| This Model is valid for Automotive grade 2 Temperature Range -40C<=Tc<=105C
| Valid for LPDDR4-4266 operation
| Part Number   VDD/VDDQ   Package   Architecture
| SCE11U64324EF-04ZA2   1.1 +0.07/-0.04  FBGA   2G bit x 32 (200b,QDP,10x14.5x1.1)
| SCE11U32322EF-04ZA2   1.1 +0.07/-0.04  FBGA   1G bit x 32 (200b,DDP,10x14.5x1.1)
[IBIS Ver]  5.0
[File Name] usesnxx32ea2.ibs
[Date]   05/20/2025
[File Rev]  1.0
[Source] Simulation of a silicon level SPICE model
[Notes]  IBIS Characteristics for I/O Buffer
  IBIS Model Revision History: Rev 2.0:
  2026-03-27 - IBIS model file PN number change
[Disclaimer]  The IBIS models are for modeling purpose only and are subject to change without any notice. UniIC is not
  responsible for any problems the models may cause.
[Copyright] Copyright 2025 UniIC Semiconductors Corp. All rights reserved
|   Component SCE11U64324EF-04ZA2
[Component] SCE11U64324EF-04ZA2
[Manufacturer] UniIC Semiconductors Corp.
[Package]
|   typ   min   max
R_pkg   1781.0m   683.00m   3347.0m
L_pkg   3.313nH   1.222nH   6.060nH
C_pkg   1.150pF   0.604pF   2.030pF
[Pin] signal_name  model_name   R_pin   L_pin   C_pin
A1   DNU   NC
A2   DNU   NC
A3   VSS   GND
A4   VDD2   POWER
A5   ZQ0   NC
A8   ZQ1   NC
A9   VDD2   POWER
A10   VSS   GND
A11   DNU   NC
A12   DNU   NC
B1   DNU   NC
B2   DQ0_A   DQ   892.22m   1.783nH   0.667pF
B3   VDDQ   POWER
B4   DQ7_A   DQ   942.05m   1.831nH   0.712pF
B5   VDDQ   POWER
B8   VDDQ   POWER
B9   DQ15_A   DQ   905.71m   1.724nH   0.652pF
B10   VDDQ   POWER
B11   DQ8_A   DQ   951.20m   1.847nH   0.708pF
B12   DNU   NC
C1   VSS   GND
C2   DQ1_A   DQ   869.40m   1.675nH   0.663pF
C3   DMI0_A   DQ   802.20m   1.539nH   0.644pF
C4   DQ6_A   DQ   695.07m   1.386nH   0.604pF
C5   VSS   GND
C8   VSS   GND
C9   DQ14_A   DQ   809.80m   1.568nH   0.657pF
C10   DMI1_A   DQ   843.49m   1.585nH   0.669pF
C11   DQ9_A   DQ   862.40m   1.663nH   0.667pF
C12   VSS   GND
D1   VDDQ   POWER
D2   VSS   GND
D3   DQS0_t_A   DQS   872.77m   1.603nH   0.663pF
D4   VSS   GND
D5   VDDQ   POWER
D8   VDDQ   POWER
D9   VSS   GND
D10   DQS1_t_A   DQS   906.95m   1.659nH   0.687pF
D11   VSS   GND
D12   VDDQ   POWER
E1   VSS   GND
E2   DQ2_A   DQ   766.79m   1.410nH   0.641pF
E3   DQS0_c_A   DQS   892.70m   1.616nH   0.682pF
E4   DQ5_A   DQ   683.10m   1.243nH   0.617pF
E5   VSS   GND
E8   VSS   GND
E9   DQ13_A   DQ   751.68m   1.328nH   0.636pF
E10   DQS1_c_A   DQS   932.00m   1.697nH   0.709pF
E11   DQ10_A   DQ   805.68m   1.499nH   0.658pF
E12   VSS   GND
F1   VDD1   POWER
F2   DQ3_A   DQ   815.20m   1.487nH   0.658pF
F3   VDDQ   POWER
F4   DQ4_A   DQ   684.70m   1.222nH   0.624pF
F5   VDD2   POWER
F8   VDD2   POWER
F9   DQ12_A   DQ   754.00m   1.333nH   0.665pF
F10   VDDQ   POWER
F11   DQ11_A   DQ   816.75m   1.527nH   0.656pF
F12   VDD1   POWER
G1   VSS   GND
G2   ODT_CA_A   ODTCA_INPUT   3223.0m   5.380nH   0.839pF
G3   VSS   GND
G4   VDD1   POWER
G5   VSS   GND
G8   VSS   GND
G9   VDD1   POWER
G10   VSS   GND
G11   NC   NC
G12   VSS   GND
H1   VDD2   POWER
H2   CA0_A   CA_INPUT   1381.0m   2.440nH   0.952pF
H3   CS1_A   CS_INPUT
H4   CS0_A   CS_INPUT
H5   VDD2   POWER
H8   VDD2   POWER
H9   CA2_A   CA_INPUT   1146.0m   2.055nH   0.856pF
H10   CA3_A   CA_INPUT   1283.0m   2.280nH   0.920pF
H11   CA4_A   CA_INPUT   1456.0m   2.590nH   1.005pF
H12   VDD2   POWER
J1   VSS   GND
J2   CA1_A   CA_INPUT   1531.0m   2.640nH   1.061pF
J3   VSS   GND
J4   CKE0_A   CKE_INPUT
J5   CKE1_A   CKE_INPUT
J8   CK_t_A   CLK_INPUT   1327.0m   2.423nH   0.917pF
J9   CK_c_A   CLK_INPUT   1352.0m   2.460nH   0.936pF
J10   VSS   GND
J11   CA5_A   CA_INPUT   1682.0m   2.901nH   1.080pF
J12   VSS   GND
K1   VDD2   POWER
K2   VSS   GND
K3   VDD2   POWER
K4   VSS   GND
K5   NC   NC
K8   NC   NC
K9   VSS   GND
K10   VDD2   POWER
K11   VSS   GND
K12   VDD2   POWER
N1   VDD2   POWER
N2   VSS   GND
N3   VDD2   POWER
N4   VSS   GND
N5   NC   NC
N8   NC   NC
N9   VSS   GND
N10   VDD2   POWER
N11   VSS   GND
N12   VDD2   POWER
P1   VSS   GND
P2   CA1_B   CA_INPUT   2001.0m   3.590nH   1.240pF
P3   VSS   GND
P4   CKE0_B   CKE_INPUT
P5   CKE1_B   CKE_INPUT
P8   CK_t_B   CLK_INPUT   1908.0m   3.371nH   1.215pF
P9   CK_c_B   CLK_INPUT   1352.0m   2.464nH   0.936pF
P10   VSS   GND
P11   CA5_B   CA_INPUT   1935.0m   3.552nH   1.192pF
P12   VSS   GND
R1   VDD2   POWER
R2   CA0_B   CA_INPUT   2110.0m   3.790nH   1.283pF
R3   CS1_B   CS_INPUT
R4   CS0_B   CS_INPUT
R5   VDD2   POWER
R8   VDD2   POWER
R9   CA2_B   CA_INPUT   1965.0m   3.398nH   1.229pF
R10   CA3_B   CA_INPUT   2061.0m   3.706nH   1.260pF
R11   CA4_B   CA_INPUT   1859.0m   3.388nH   1.151pF
R12   VDD2   POWER
T1   VSS   GND
T2   ODT_CA_B   ODTCA_INPUT   1974.0m   3.548nH   1.128pF
T3   VSS   GND
T4   VDD1   POWER
T5   VSS   GND
T8   VSS   GND
T9   VDD1   POWER
T10   VSS   GND
T11   RESET_n   NC
T12   VSS   GND
U1   VDD1   POWER
U2   DQ3_B   DQ   2687.0m   4.766nH   1.558pF
U3   VDDQ   POWER
U4   DQ4_B   DQ   2425.0m   4.233nH   1.469pF
U5   VDD2   POWER
U8   VDD2   POWER
U9   DQ12_B   DQ   3116.0m   5.207nH   1.812pF
U10   VDDQ   POWER
U11   DQ11_B   DQ   3179.0m   5.321nH   1.828pF
U12   VDD1   POWER
V1   VSS   GND
V2   DQ2_B   DQ   2588.0m   4.551nH   1.513pF
V3   DQS0_c_B   DQS   2438.0m   4.346nH   1.466pF
V4   DQ5_B   DQ   2290.0m   4.012nH   1.391pF
V5   VSS   GND
V8   VSS   GND
V9   DQ13_B   DQ   3013.0m   5.038nH   1.759pF
V10   DQS1_c_B   DQS   3073.0m   5.198nH   1.833pF
V11   DQ10_B   DQ   3240.0m   5.404nH   1.898pF
V12   VSS   GND
W1   VDDQ   POWER
W2   VSS   GND
W3   DQS0_t_B   DQS   2438.0m   4.346nH   1.466pF
W4   VSS   GND
W5   VDDQ   POWER
W8   VDDQ   POWER
W9   VSS   GND
W10   DQS1_t_B   DQS   3167.0m   5.386nH   1.871pF
W11   VSS   GND
W12   VDDQ   POWER
Y1   VSS   GND
Y2   DQ1_B   DQ   2484.0m   4.410nH   1.467pF
Y3   DMI0_B   DQ   2282.0m   4.056nH   1.378pF
Y4   DQ6_B   DQ   2149.0m   3.822nH   1.313pF
Y5   VSS   GND
Y8   VSS   GND
Y9   DQ14_B   DQ   3051.0m   5.183nH   1.804pF
Y10   DMI1_B   DQ   3195.0m   5.155nH   1.899pF
Y11   DQ9_B   DQ   3347.0m   5.680nH   1.932pF
Y12   VSS   GND
AA1   DNU   NC
AA2   DQ0_B   DQ   2472.0m   4.484nH   1.453pF
AA3   VDDQ   POWER
AA4   DQ7_B   DQ   2196.0m   4.004nH   1.284pF
AA5   VDDQ   POWER
AA8   VDDQ   POWER
AA9   DQ15_B   DQ   3046.0m   5.081nH   1.820pF
AA10  VDDQ   POWER
AA11  DQ8_B   DQ   3565.0m   6.060nH   2.037pF
AA12  DNU   NC
AB1   DNU   NC
AB2   DNU   NC
AB3   VSS   GND
AB4   VDD2   POWER
AB5   VSS   GND
AB8   VSS   GND
AB9   VDD2   POWER
AB10  VSS   GND
AB11  DNU   NC
AB12  DNU   NC
[Diff Pin]  inv_pin  vdiff   tdelay_typ   tdelay_min   tdelay_max
D3   E3   0.120V   0.000s   NA   NA
W3   V3   0.120V   0.000s   NA   NA
D10   E10   0.120V   0.000s   NA   NA
W10   V10   0.120V   0.000s   NA   NA
J8   J9   0.145V   0.000s   NA   NA
P8   P9   0.145V   0.000s   NA   NA
|   Component SCE11U32322EF-04ZA2
[Component] SCE11U32322EF-04ZA2
[Manufacturer] UniIC Semiconductors Corp.
[Package]
|   typ   min   max
R_pkg   1781.0m   683.00m   3340.0m
L_pkg   3.313nH   1.222nH   6.060nH
C_pkg   1.150pF   0.604pF   2.030pF
[Pin] signal_name  model_name   R_pin   L_pin   C_pin
A1   DNU   NC
A2   DNU   NC
A3   VSS   GND
A4   VDD2   POWER
A5   ZQ0   NC
A8   ZQ1   NC
A9   VDD2   POWER
A10   VSS   GND
A11   DNU   NC
A12   DNU   NC
B1   DNU   NC
B2   DQ0_A   DQ   892.22m   1.783nH   0.667pF
B3   VDDQ   POWER
B4   DQ7_A   DQ   942.05m   1.831nH   0.712pF
B5   VDDQ   POWER
B8   VDDQ   POWER
B9   DQ15_A   DQ   905.71m   1.724nH   0.652pF
B10   VDDQ   POWER
B11   DQ8_A   DQ   951.20m   1.847nH   0.708pF
B12   DNU   NC
C1   VSS   GND
C2   DQ1_A   DQ   869.40m   1.675nH   0.663pF
C3   DMI0_A   DQ   802.20m   1.539nH   0.644pF
C4   DQ6_A   DQ   695.07m   1.386nH   0.604pF
C5   VSS   GND
C8   VSS   GND
C9   DQ14_A   DQ   809.80m   1.568nH   0.657pF
C10   DMI1_A   DQ   843.49m   1.585nH   0.669pF
C11   DQ9_A   DQ   862.40m   1.663nH   0.667pF
C12   VSS   GND
D1   VDDQ   POWER
D2   VSS   GND
D3   DQS0_t_A   DQS   872.77m   1.603nH   0.663pF
D4   VSS   GND
D5   VDDQ   POWER
D8   VDDQ   POWER
D9   VSS   GND
D10   DQS1_t_A   DQS   906.95m   1.659nH   0.687pF
D11   VSS   GND
D12   VDDQ   POWER
E1   VSS   GND
E2   DQ2_A   DQ   766.79m   1.410nH   0.641pF
E3   DQS0_c_A   DQS   892.70m   1.616nH   0.682pF
E4   DQ5_A   DQ   683.10m   1.243nH   0.617pF
E5   VSS   GND
E8   VSS   GND
E9   DQ13_A   DQ   751.68m   1.328nH   0.636pF
E10   DQS1_c_A   DQS   932.00m   1.697nH   0.709pF
E11   DQ10_A   DQ   805.68m   1.499nH   0.658pF
E12   VSS   GND
F1   VDD1   POWER
F2   DQ3_A   DQ   815.20m   1.487nH   0.658pF
F3   VDDQ   POWER
F4   DQ4_A   DQ   684.70m   1.222nH   0.624pF
F5   VDD2   POWER
F8   VDD2   POWER
F9   DQ12_A   DQ   754.00m   1.333nH   0.665pF
F10   VDDQ   POWER
F11   DQ11_A   DQ   816.75m   1.527nH   0.656pF
F12   VDD1   POWER
G1   VSS   GND
G2   ODT_CA_A   ODTCA_INPUT   3223.0m   5.380nH   0.839pF
G3   VSS   GND
G4   VDD1   POWER
G5   VSS   GND
G8   VSS   GND
G9   VDD1   POWER
G10   VSS   GND
G11   NC   NC
G12   VSS   GND
H1   VDD2   POWER
H2   CA0_A   CA_INPUT   1381.0m   2.440nH   0.952pF
H3   NC   NC
H4   CS0_A   CS_INPUT
H5   VDD2   POWER
H8   VDD2   POWER
H9   CA2_A   CA_INPUT   1146.0m   2.055nH   0.856pF
H10   CA3_A   CA_INPUT   1283.0m   2.280nH   0.920pF
H11   CA4_A   CA_INPUT   1456.0m   2.590nH   1.005pF
H12   VDD2   POWER
J1   VSS   GND
J2   CA1_A   CA_INPUT   1531.0m   2.640nH   1.061pF
J3   VSS   GND
J4   CKE0_A   CKE_INPUT
J5   NC   NC
J8   CK_t_A   CLK_INPUT   1327.0m   2.423nH   0.917pF
J9   CK_c_A   CLK_INPUT   1352.0m   2.460nH   0.936pF
J10   VSS   GND
J11   CA5_A   CA_INPUT   1682.0m   2.901nH   1.080pF
J12   VSS   GND
K1   VDD2   POWER
K2   VSS   GND
K3   VDD2   POWER
K4   VSS   GND
K5   NC   NC
K8   NC   NC
K9   VSS   GND
K10   VDD2   POWER
K11   VSS   GND
K12   VDD2   POWER
N1   VDD2   POWER
N2   VSS   GND
N3   VDD2   POWER
N4   VSS   GND
N5   NC   NC
N8   NC   NC
N9   VSS   GND
N10   VDD2   POWER
N11   VSS   GND
N12   VDD2   POWER
P1   VSS   GND
P2   CA1_B   CA_INPUT   2001.0m   3.590nH   1.240pF
P3   VSS   GND
P4   CKE0_B   CKE_INPUT
P5   NC   NC
P8   CK_t_B   CLK_INPUT   1908.0m   3.371nH   1.215pF
P9   CK_c_B   CLK_INPUT   1352.0m   2.464nH   0.936pF
P10   VSS   GND
P11   CA5_B   CA_INPUT   1935.0m   3.552nH   1.192pF
P12   VSS   GND
R1   VDD2   POWER
R2   CA0_B   CA_INPUT   2110.0m   3.790nH   1.283pF
R3   NC   NC
R4   CS0_B   CS_INPUT
R5   VDD2   POWER
R8   VDD2   POWER
R9   CA2_B   CA_INPUT   1965.0m   3.398nH   1.229pF
R10   CA3_B   CA_INPUT   2061.0m   3.706nH   1.260pF
R11   CA4_B   CA_INPUT   1859.0m   3.388nH   1.151pF
R12   VDD2   POWER
T1   VSS   GND
T2   ODT_CA_B   ODTCA_INPUT   1974.0m   3.548nH   1.128pF
T3   VSS   GND
T4   VDD1   POWER
T5   VSS   GND
T8   VSS   GND
T9   VDD1   POWER
T10   VSS   GND
T11   RESET_n   NC
T12   VSS   GND
U1   VDD1   POWER
U2   DQ3_B   DQ   2687.0m   4.766nH   1.558pF
U3   VDDQ   POWER
U4   DQ4_B   DQ   2425.0m   4.233nH   1.469pF
U5   VDD2   POWER
U8   VDD2   POWER
U9   DQ12_B   DQ   3116.0m   5.207nH   1.812pF
U10   VDDQ   POWER
U11   DQ11_B   DQ   3179.0m   5.321nH   1.828pF
U12   VDD1   POWER
V1   VSS   GND
V2   DQ2_B   DQ   2588.0m   4.551nH   1.513pF
V3   DQS0_c_B   DQS   2438.0m   4.346nH   1.466pF
V4   DQ5_B   DQ   2290.0m   4.012nH   1.391pF
V5   VSS   GND
V8   VSS   GND
V9   DQ13_B   DQ   3013.0m   5.038nH   1.759pF
V10   DQS1_c_B   DQS   3073.0m   5.198nH   1.833pF
V11   DQ10_B   DQ   3240.0m   5.404nH   1.898pF
V12   VSS   GND
W1   VDDQ   POWER
W2   VSS   GND
W3   DQS0_t_B   DQS   2438.0m   4.346nH   1.466pF
W4   VSS   GND
W5   VDDQ   POWER
W8   VDDQ   POWER
W9   VSS   GND
W10   DQS1_t_B   DQS   3167.0m   5.386nH   1.871pF
W11   VSS   GND
W12   VDDQ   POWER
Y1   VSS   GND
Y2   DQ1_B   DQ   2484.0m   4.410nH   1.467pF
Y3   DMI0_B   DQ   2282.0m   4.056nH   1.378pF
Y4   DQ6_B   DQ   2149.0m   3.822nH   1.313pF
Y5   VSS   GND
Y8   VSS   GND
Y9   DQ14_B   DQ   3051.0m   5.183nH   1.804pF
Y10   DMI1_B   DQ   3195.0m   5.155nH   1.899pF
Y11   DQ9_B   DQ   3347.0m   5.680nH   1.932pF
Y12   VSS   GND
AA1   DNU   NC
AA2   DQ0_B   DQ   2472.0m   4.484nH   1.453pF
AA3   VDDQ   POWER
AA4   DQ7_B   DQ   2196.0m   4.004nH   1.284pF
AA5   VDDQ   POWER
AA8   VDDQ   POWER
AA9   DQ15_B   DQ   3046.0m   5.081nH   1.820pF
AA10  VDDQ   POWER
AA11  DQ8_B   DQ   356.05m   6.060nH   2.037pF
AA12  DNU   NC
AB1   DNU   NC
AB2   DNU   NC
AB3   VSS   GND
AB4   VDD2   POWER
AB5   VSS   GND
AB8   VSS   GND
AB9   VDD2   POWER
AB10  VSS   GND
AB11  DNU   NC
AB12  DNU   NC
[Diff Pin]  inv_pin  vdiff   tdelay_typ   tdelay_min   tdelay_max
D3   E3   0.120V   0.000s   NA   NA
W3   V3   0.120V   0.000s   NA   NA
D10   E10   0.120V   0.000s   NA   NA
W10   V10   0.120V   0.000s   NA   NA
J8   J9   0.145V   0.000s   NA   NA
P8   P9   0.145V   0.000s   NA   NA
|   Model Selector
[Model Selector] DQ
| Data I/O models
DQ_PD40_SOC-ODT40_VOH30_4266   40 Ohm Pulldown, 40 Ohm System ODT Setting, VOH=VDDQ/3.0, 3200-4266Mbps
DQ_PD40_SOC-ODT48_VOH30_4266   40 Ohm Pulldown, 48 Ohm System ODT Setting, VOH=VDDQ/3.0, 3200-4266Mbps
DQ_PD40_SOC-ODT60_VOH30_4266   40 Ohm Pulldown, 60 Ohm System ODT Setting, VOH=VDDQ/3.0, 3200-4266Mbps
DQ_PD40_SOC-ODT80_VOH30_4266   40 Ohm Pulldown, 80 Ohm System ODT Setting, VOH=VDDQ/3.0, 3200-4266Mbps
DQ_PD40_SOC-ODT120_VOH30_4266   40 Ohm Pulldown, 120 Ohm System ODT Setting, VOH=VDDQ/3.0, 3200-4266Mbps
DQ_PD40_SOC-ODT240_VOH30_4266   40 Ohm Pulldown, 240 Ohm System ODT Setting, VOH=VDDQ/3.0, 3200-4266Mbps
DQ_PD40_SOC-ODTDIS_VOH30_4266   40 Ohm Pulldown, SOC ODT disabled setting, VOH=VDDQ/3.0 cal. point, 3200-4266Mbps
DQ_PD40_SOC-ODT80_VOH25_4266   40 Ohm Pulldown, 80 Ohm System ODT Setting, VOH=VDDQ/2.5, 3200-4266Mbps
DQ_PD40_SOC-ODT120_VOH25_4266   40 Ohm Pulldown, 120 Ohm System ODT Setting, VOH=VDDQ/2.5, 3200-4266Mbps
DQ_PD40_SOC-ODT240_VOH25_4266   40 Ohm Pulldown, 240 Ohm System ODT Setting, VOH=VDDQ/2.5, 3200-4266Mbps
DQ_PD40_SOC-ODTDIS_VOH25_4266   40 Ohm Pulldown, SOC ODT disabled setting, VOH=VDDQ/2.5 cal. point, 3200-4266Mbps
DQ_PD48_SOC-ODT40_VOH30_4266   48 Ohm Pulldown, 40 Ohm System ODT Setting, VOH=VDDQ/3.0, 3200-4266Mbps
DQ_PD48_SOC-ODT48_VOH30_4266   48 Ohm Pulldown, 48 Ohm System ODT Setting, VOH=VDDQ/3.0, 3200-4266Mbps
DQ_PD48_SOC-ODT60_VOH30_4266   48 Ohm Pulldown, 60 Ohm System ODT Setting, VOH=VDDQ/3.0, 3200-4266Mbps
DQ_PD48_SOC-ODT80_VOH30_4266   48 Ohm Pulldown, 80 Ohm System ODT Setting, VOH=VDDQ/3.0, 3200-4266Mbps
DQ_PD48_SOC-ODT120_VOH30_4266   48 Ohm Pulldown, 120 Ohm System ODT Setting, VOH=VDDQ/3.0, 3200-4266Mbps
DQ_PD48_SOC-ODT240_VOH30_4266   48 Ohm Pulldown, 240 Ohm System ODT Setting, VOH=VDDQ/3.0, 3200-4266Mbps
DQ_PD48_SOC-ODTDIS_VOH30_4266   48 Ohm Pulldown, SOC ODT disabled setting, VOH=VDDQ/3.0 cal. point, 3200-4266Mbps
DQ_PD48_SOC-ODT80_VOH25_4266   48 Ohm Pulldown, 80 Ohm System ODT Setting, VOH=VDDQ/2.5, 3200-4266Mbps
DQ_PD48_SOC-ODT120_VOH25_4266   48 Ohm Pulldown, 120 Ohm System ODT Setting, VOH=VDDQ/2.5, 3200-4266Mbps
DQ_PD48_SOC-ODT240_VOH25_4266   48 Ohm Pulldown, 240 Ohm System ODT Setting, VOH=VDDQ/2.5, 3200-4266Mbps
DQ_PD48_SOC-ODTDIS_VOH25_4266   48 Ohm Pulldown, SOC ODT disabled setting, VOH=VDDQ/2.5 cal. point, 3200-4266Mbps
DQ_PD60_SOC-ODT40_VOH30_4266   60 Ohm Pulldown, 40 Ohm System ODT Setting, VOH=VDDQ/3.0, 3200-4266Mbps
DQ_PD60_SOC-ODT48_VOH30_4266   60 Ohm Pulldown, 48 Ohm System ODT Setting, VOH=VDDQ/3.0, 3200-4266Mbps
DQ_PD60_SOC-ODT60_VOH30_4266   60 Ohm Pulldown, 60 Ohm System ODT Setting, VOH=VDDQ/3.0, 3200-4266Mbps
DQ_PD60_SOC-ODT80_VOH30_4266   60 Ohm Pulldown, 80 Ohm System ODT Setting, VOH=VDDQ/3.0, 3200-4266Mbps
DQ_PD60_SOC-ODT120_VOH30_4266   60 Ohm Pulldown, 120 Ohm System ODT Setting, VOH=VDDQ/3.0, 3200-4266Mbps
DQ_PD60_SOC-ODT240_VOH30_4266   60 Ohm Pulldown, 240 Ohm System ODT Setting, VOH=VDDQ/3.0, 3200-4266Mbps
DQ_PD60_SOC-ODTDIS_VOH30_4266   60 Ohm Pulldown, SOC ODT disabled setting, VOH=VDDQ/3.0 cal. point, 3200-4266Mbps
DQ_PD60_SOC-ODT80_VOH25_4266   60 Ohm Pulldown, 80 Ohm System ODT Setting, VOH=VDDQ/2.5, 3200-4266Mbps
DQ_PD60_SOC-ODT120_VOH25_4266   60 Ohm Pulldown, 120 Ohm System ODT Setting, VOH=VDDQ/2.5, 3200-4266Mbps
DQ_PD60_SOC-ODT240_VOH25_4266   60 Ohm Pulldown, 240 Ohm System ODT Setting, VOH=VDDQ/2.5, 3200-4266Mbps
DQ_PD60_SOC-ODTDIS_VOH25_4266   60 Ohm Pulldown, SOC ODT disabled setting, VOH=VDDQ/2.5 cal. point, 3200-4266Mbps
DQ_PD80_SOC-ODT40_VOH30_4266   80 Ohm Pulldown, 40 Ohm System ODT Setting, VOH=VDDQ/3.0, 3200-4266Mbps
DQ_PD80_SOC-ODT48_VOH30_4266   80 Ohm Pulldown, 48 Ohm System ODT Setting, VOH=VDDQ/3.0, 3200-4266Mbps
DQ_PD80_SOC-ODT60_VOH30_4266   80 Ohm Pulldown, 60 Ohm System ODT Setting, VOH=VDDQ/3.0, 3200-4266Mbps
DQ_PD80_SOC-ODT80_VOH30_4266   80 Ohm Pulldown, 80 Ohm System ODT Setting, VOH=VDDQ/3.0, 3200-4266Mbps
DQ_PD80_SOC-ODT120_VOH30_4266   80 Ohm Pulldown, 120 Ohm System ODT Setting, VOH=VDDQ/3.0, 3200-4266Mbps
DQ_PD80_SOC-ODT240_VOH30_4266   80 Ohm Pulldown, 240 Ohm System ODT Setting, VOH=VDDQ/3.0, 3200-4266Mbps
DQ_PD80_SOC-ODTDIS_VOH30_4266   80 Ohm Pulldown, SOC ODT disabled setting, VOH=VDDQ/3.0 cal. point, 3200-4266Mbps
DQ_PD80_SOC-ODT80_VOH25_4266   80 Ohm Pulldown, 80 Ohm System ODT Setting, VOH=VDDQ/2.5, 3200-4266Mbps
DQ_PD80_SOC-ODT120_VOH25_4266   80 Ohm Pulldown, 120 Ohm System ODT Setting, VOH=VDDQ/2.5, 3200-4266Mbps
DQ_PD80_SOC-ODT240_VOH25_4266   80 Ohm Pulldown, 240 Ohm System ODT Setting, VOH=VDDQ/2.5, 3200-4266Mbps
DQ_PD80_SOC-ODTDIS_VOH25_4266   80 Ohm Pulldown, SOC ODT disabled setting, VOH=VDDQ/2.5 cal. point, 3200-4266Mbps
DQ_PD120_SOC-ODT40_VOH30_4266   120 Ohm Pulldown, 40 Ohm System ODT Setting, VOH=VDDQ/3.0, 3200-4266Mbps
DQ_PD120_SOC-ODT48_VOH30_4266   120 Ohm Pulldown, 48 Ohm System ODT Setting, VOH=VDDQ/3.0, 3200-4266Mbps
DQ_PD120_SOC-ODT60_VOH30_4266   120 Ohm Pulldown, 60 Ohm System ODT Setting, VOH=VDDQ/3.0, 3200-4266Mbps
DQ_PD120_SOC-ODT80_VOH30_4266   120 Ohm Pulldown, 80 Ohm System ODT Setting, VOH=VDDQ/3.0, 3200-4266Mbps
DQ_PD120_SOC-ODT120_VOH30_4266  120 Ohm Pulldown, 120 Ohm System ODT Setting, VOH=VDDQ/3.0, 3200-4266Mbps
DQ_PD120_SOC-ODT240_VOH30_4266  120 Ohm Pulldown, 240 Ohm System ODT Setting, VOH=VDDQ/3.0, 3200-4266Mbps
DQ_PD120_SOC-ODTDIS_VOH30_4266  120 Ohm Pulldown, SOC ODT disabled setting, VOH=VDDQ/3.0 cal. point, 3200-4266Mbps
DQ_PD120_SOC-ODT80_VOH25_4266   120 Ohm Pulldown, 80 Ohm System ODT Setting, VOH=VDDQ/2.5, 3200-4266Mbps
DQ_PD120_SOC-ODT120_VOH25_4266  120 Ohm Pulldown, 120 Ohm System ODT Setting, VOH=VDDQ/2.5, 3200-4266Mbps
DQ_PD120_SOC-ODT240_VOH25_4266  120 Ohm Pulldown, 240 Ohm System ODT Setting, VOH=VDDQ/2.5, 3200-4266Mbps
DQ_PD120_SOC-ODTDIS_VOH25_4266  120 Ohm Pulldown, SOC ODT disabled setting, VOH=VDDQ/2.5 cal. point, 3200-4266Mbps
DQ_PD240_SOC-ODT40_VOH30_4266   240 Ohm Pulldown, 40 Ohm System ODT Setting, VOH=VDDQ/3.0, 3200-4266Mbps
DQ_PD240_SOC-ODT48_VOH30_4266   240 Ohm Pulldown, 48 Ohm System ODT Setting, VOH=VDDQ/3.0, 3200-4266Mbps
DQ_PD240_SOC-ODT60_VOH30_4266   240 Ohm Pulldown, 60 Ohm System ODT Setting, VOH=VDDQ/3.0, 3200-4266Mbps
DQ_PD240_SOC-ODT80_VOH30_4266   240 Ohm Pulldown, 80 Ohm System ODT Setting, VOH=VDDQ/3.0, 3200-4266Mbps
DQ_PD240_SOC-ODT120_VOH30_4266  240 Ohm Pulldown, 120 Ohm System ODT Setting, VOH=VDDQ/3.0, 3200-4266Mbps
DQ_PD240_SOC-ODT240_VOH30_4266  240 Ohm Pulldown, 240 Ohm System ODT Setting, VOH=VDDQ/3.0, 3200-4266Mbps
DQ_PD240_SOC-ODTDIS_VOH30_4266  240 Ohm Pulldown, SOC ODT disabled setting, VOH=VDDQ/3.0 cal. point, 3200-4266Mbps
DQ_PD240_SOC-ODT80_VOH25_4266   240 Ohm Pulldown, 80 Ohm System ODT Setting, VOH=VDDQ/2.5, 3200-4266Mbps
DQ_PD240_SOC-ODT120_VOH25_4266  240 Ohm Pulldown, 120 Ohm System ODT Setting, VOH=VDDQ/2.5, 3200-4266Mbps
DQ_PD240_SOC-ODT240_VOH25_4266  240 Ohm Pulldown, 240 Ohm System ODT Setting, VOH=VDDQ/2.5, 3200-4266Mbps
DQ_PD240_SOC-ODTDIS_VOH25_4266  240 Ohm Pulldown, SOC ODT disabled setting, VOH=VDDQ/2.5 cal. point, 3200-4266Mbps
DQ_IN_ODTOFF_4266   with no ODT, 3200-4266Mbps
DQ_IN_ODT40_4266   with 40ohm ODT, 3200-4266Mbps
DQ_IN_ODT48_4266   with 48ohm ODT, 3200-4266Mbps
DQ_IN_ODT60_4266   with 60ohm ODT, 3200-4266Mbps
DQ_IN_ODT80_4266   with 80ohm ODT, 3200-4266Mbps
DQ_IN_ODT120_4266   with 120ohm ODT, 3200-4266Mbps
DQ_IN_ODT240_4266   with 240ohm ODT, 3200-4266Mbps
[Model Selector] DQS
| Data Strobe I/O models
DQS_PD40_SOC-ODT40_VOH30_4266   40 Ohm Pulldown, 40 Ohm System ODT Setting, VOH=VDDQ/3.0, 3200-4266Mbps
DQS_PD40_SOC-ODT48_VOH30_4266   40 Ohm Pulldown, 48 Ohm System ODT Setting, VOH=VDDQ/3.0, 3200-4266Mbps
DQS_PD40_SOC-ODT60_VOH30_4266   40 Ohm Pulldown, 60 Ohm System ODT Setting, VOH=VDDQ/3.0, 3200-4266Mbps
DQS_PD40_SOC-ODT80_VOH30_4266   40 Ohm Pulldown, 80 Ohm System ODT Setting, VOH=VDDQ/3.0, 3200-4266Mbps
DQS_PD40_SOC-ODT120_VOH30_4266  40 Ohm Pulldown, 120 Ohm System ODT Setting, VOH=VDDQ/3.0, 3200-4266Mbps
DQS_PD40_SOC-ODT240_VOH30_4266  40 Ohm Pulldown, 240 Ohm System ODT Setting, VOH=VDDQ/3.0, 3200-4266Mbps
DQS_PD40_SOC-ODTDIS_VOH30_4266  40 Ohm Pulldown, SOC ODT disabled setting, VOH=VDDQ/3.0 cal. point, 3200-4266Mbps
DQS_PD40_SOC-ODT80_VOH25_4266   40 Ohm Pulldown, 80 Ohm System ODT Setting, VOH=VDDQ/2.5, 3200-4266Mbps
DQS_PD40_SOC-ODT120_VOH25_4266  40 Ohm Pulldown, 120 Ohm System ODT Setting, VOH=VDDQ/2.5, 3200-4266Mbps
DQS_PD40_SOC-ODT240_VOH25_4266  40 Ohm Pulldown, 240 Ohm System ODT Setting, VOH=VDDQ/2.5, 3200-4266Mbps
DQS_PD40_SOC-ODTDIS_VOH25_4266  40 Ohm Pulldown, SOC ODT disabled setting, VOH=VDDQ/2.5 cal. point, 3200-4266Mbps
DQS_PD48_SOC-ODT40_VOH30_4266   48 Ohm Pulldown, 40 Ohm System ODT Setting, VOH=VDDQ/3.0, 3200-4266Mbps
DQS_PD48_SOC-ODT48_VOH30_4266   48 Ohm Pulldown, 48 Ohm System ODT Setting, VOH=VDDQ/3.0, 3200-4266Mbps
DQS_PD48_SOC-ODT60_VOH30_4266   48 Ohm Pulldown, 60 Ohm System ODT Setting, VOH=VDDQ/3.0, 3200-4266Mbps
DQS_PD48_SOC-ODT80_VOH30_4266   48 Ohm Pulldown, 80 Ohm System ODT Setting, VOH=VDDQ/3.0, 3200-4266Mbps
DQS_PD48_SOC-ODT120_VOH30_4266  48 Ohm Pulldown, 120 Ohm System ODT Setting, VOH=VDDQ/3.0, 3200-4266Mbps
DQS_PD48_SOC-ODT240_VOH30_4266  48 Ohm Pulldown, 240 Ohm System ODT Setting, VOH=VDDQ/3.0, 3200-4266Mbps
DQS_PD48_SOC-ODTDIS_VOH30_4266  48 Ohm Pulldown, SOC ODT disabled setting, VOH=VDDQ/3.0 cal. point, 3200-4266Mbps
DQS_PD48_SOC-ODT80_VOH25_4266   48 Ohm Pulldown, 80 Ohm System ODT Setting, VOH=VDDQ/2.5, 3200-4266Mbps
DQS_PD48_SOC-ODT120_VOH25_4266  48 Ohm Pulldown, 120 Ohm System ODT Setting, VOH=VDDQ/2.5, 3200-4266Mbps
DQS_PD48_SOC-ODT240_VOH25_4266  48 Ohm Pulldown, 240 Ohm System ODT Setting, VOH=VDDQ/2.5, 3200-4266Mbps
DQS_PD48_SOC-ODTDIS_VOH25_4266  48 Ohm Pulldown, SOC ODT disabled setting, VOH=VDDQ/2.5 cal. point, 3200-4266Mbps
DQS_PD60_SOC-ODT40_VOH30_4266   60 Ohm Pulldown, 40 Ohm System ODT Setting, VOH=VDDQ/3.0, 3200-4266Mbps
DQS_PD60_SOC-ODT48_VOH30_4266   60 Ohm Pulldown, 48 Ohm System ODT Setting, VOH=VDDQ/3.0, 3200-4266Mbps
DQS_PD60_SOC-ODT60_VOH30_4266   60 Ohm Pulldown, 60 Ohm System ODT Setting, VOH=VDDQ/3.0, 3200-4266Mbps
DQS_PD60_SOC-ODT80_VOH30_4266   60 Ohm Pulldown, 80 Ohm System ODT Setting, VOH=VDDQ/3.0, 3200-4266Mbps
DQS_PD60_SOC-ODT120_VOH30_4266  60 Ohm Pulldown, 120 Ohm System ODT Setting, VOH=VDDQ/3.0, 3200-4266Mbps
DQS_PD60_SOC-ODT240_VOH30_4266  60 Ohm Pulldown, 240 Ohm System ODT Setting, VOH=VDDQ/3.0, 3200-4266Mbps
DQS_PD60_SOC-ODTDIS_VOH30_4266  60 Ohm Pulldown, SOC ODT disabled setting, VOH=VDDQ/3.0 cal. point, 3200-4266Mbps
DQS_PD60_SOC-ODT80_VOH25_4266   60 Ohm Pulldown, 80 Ohm System ODT Setting, VOH=VDDQ/2.5, 3200-4266Mbps
DQS_PD60_SOC-ODT120_VOH25_4266  60 Ohm Pulldown, 120 Ohm System ODT Setting, VOH=VDDQ/2.5, 3200-4266Mbps
DQS_PD60_SOC-ODT240_VOH25_4266  60 Ohm Pulldown, 240 Ohm System ODT Setting, VOH=VDDQ/2.5, 3200-4266Mbps
DQS_PD60_SOC-ODTDIS_VOH25_4266  60 Ohm Pulldown, SOC ODT disabled setting, VOH=VDDQ/2.5 cal. point, 3200-4266Mbps
DQS_PD80_SOC-ODT40_VOH30_4266   80 Ohm Pulldown, 40 Ohm System ODT Setting, VOH=VDDQ/3.0, 3200-4266Mbps
DQS_PD80_SOC-ODT48_VOH30_4266   80 Ohm Pulldown, 48 Ohm System ODT Setting, VOH=VDDQ/3.0, 3200-4266Mbps
DQS_PD80_SOC-ODT60_VOH30_4266   80 Ohm Pulldown, 60 Ohm System ODT Setting, VOH=VDDQ/3.0, 3200-4266Mbps
DQS_PD80_SOC-ODT80_VOH30_4266   80 Ohm Pulldown, 80 Ohm System ODT Setting, VOH=VDDQ/3.0, 3200-4266Mbps
DQS_PD80_SOC-ODT120_VOH30_4266  80 Ohm Pulldown, 120 Ohm System ODT Setting, VOH=VDDQ/3.0, 3200-4266Mbps
DQS_PD80_SOC-ODT240_VOH30_4266  80 Ohm Pulldown, 240 Ohm System ODT Setting, VOH=VDDQ/3.0, 3200-4266Mbps
DQS_PD80_SOC-ODTDIS_VOH30_4266  80 Ohm Pulldown, SOC ODT disabled setting, VOH=VDDQ/3.0 cal. point, 3200-4266Mbps
DQS_PD80_SOC-ODT80_VOH25_4266   80 Ohm Pulldown, 80 Ohm System ODT Setting, VOH=VDDQ/2.5, 3200-4266Mbps
DQS_PD80_SOC-ODT120_VOH25_4266  80 Ohm Pulldown, 120 Ohm System ODT Setting, VOH=VDDQ/2.5, 3200-4266Mbps
DQS_PD80_SOC-ODT240_VOH25_4266  80 Ohm Pulldown, 240 Ohm System ODT Setting, VOH=VDDQ/2.5, 3200-4266Mbps
DQS_PD80_SOC-ODTDIS_VOH25_4266  80 Ohm Pulldown, SOC ODT disabled setting, VOH=VDDQ/2.5 cal. point, 3200-4266Mbps
DQS_PD120_SOC-ODT40_VOH30_4266  120 Ohm Pulldown, 40 Ohm System ODT Setting, VOH=VDDQ/3.0, 3200-4266Mbps
DQS_PD120_SOC-ODT48_VOH30_4266  120 Ohm Pulldown, 48 Ohm System ODT Setting, VOH=VDDQ/3.0, 3200-4266Mbps
DQS_PD120_SOC-ODT60_VOH30_4266  120 Ohm Pulldown, 60 Ohm System ODT Setting, VOH=VDDQ/3.0, 3200-4266Mbps
DQS_PD120_SOC-ODT80_VOH30_4266  120 Ohm Pulldown, 80 Ohm System ODT Setting, VOH=VDDQ/3.0, 3200-4266Mbps
DQS_PD120_SOC-ODT120_VOH30_4266 120 Ohm Pulldown, 120 Ohm System ODT Setting, VOH=VDDQ/3.0, 3200-4266Mbps
DQS_PD120_SOC-ODT240_VOH30_4266 120 Ohm Pulldown, 240 Ohm System ODT Setting, VOH=VDDQ/3.0, 3200-4266Mbps
DQS_PD120_SOC-ODTDIS_VOH30_4266 120 Ohm Pulldown, SOC ODT disabled setting, VOH=VDDQ/3.0 cal. point, 3200-4266Mbps
DQS_PD120_SOC-ODT80_VOH25_4266  120 Ohm Pulldown, 80 Ohm System ODT Setting, VOH=VDDQ/2.5, 3200-4266Mbps
DQS_PD120_SOC-ODT120_VOH25_4266 120 Ohm Pulldown, 120 Ohm System ODT Setting, VOH=VDDQ/2.5, 3200-4266Mbps
DQS_PD120_SOC-ODT240_VOH25_4266 120 Ohm Pulldown, 240 Ohm System ODT Setting, VOH=VDDQ/2.5, 3200-4266Mbps
DQS_PD120_SOC-ODTDIS_VOH25_4266 120 Ohm Pulldown, SOC ODT disabled setting, VOH=VDDQ/2.5 cal. point, 3200-4266Mbps
DQS_PD240_SOC-ODT40_VOH30_4266  240 Ohm Pulldown, 40 Ohm System ODT Setting, VOH=VDDQ/3.0, 3200-4266Mbps
DQS_PD240_SOC-ODT48_VOH30_4266  240 Ohm Pulldown, 48 Ohm System ODT Setting, VOH=VDDQ/3.0, 3200-4266Mbps
DQS_PD240_SOC-ODT60_VOH30_4266  240 Ohm Pulldown, 60 Ohm System ODT Setting, VOH=VDDQ/3.0, 3200-4266Mbps
DQS_PD240_SOC-ODT80_VOH30_4266  240 Ohm Pulldown, 80 Ohm System ODT Setting, VOH=VDDQ/3.0, 3200-4266Mbps
DQS_PD240_SOC-ODT120_VOH30_4266 240 Ohm Pulldown, 120 Ohm System ODT Setting, VOH=VDDQ/3.0, 3200-4266Mbps
DQS_PD240_SOC-ODT240_VOH30_4266 240 Ohm Pulldown, 240 Ohm System ODT Setting, VOH=VDDQ/3.0, 3200-4266Mbps
DQS_PD240_SOC-ODTDIS_VOH30_4266 240 Ohm Pulldown, SOC ODT disabled setting, VOH=VDDQ/3.0 cal. point, 3200-4266Mbps
DQS_PD240_SOC-ODT80_VOH25_4266  240 Ohm Pulldown, 80 Ohm System ODT Setting, VOH=VDDQ/2.5, 3200-4266Mbps
DQS_PD240_SOC-ODT120_VOH25_4266 240 Ohm Pulldown, 120 Ohm System ODT Setting, VOH=VDDQ/2.5, 3200-4266Mbps
DQS_PD240_SOC-ODT240_VOH25_4266 240 Ohm Pulldown, 240 Ohm System ODT Setting, VOH=VDDQ/2.5, 3200-4266Mbps
DQS_PD240_SOC-ODTDIS_VOH25_4266 240 Ohm Pulldown, SOC ODT disabled setting, VOH=VDDQ/2.5 cal. point, 3200-4266Mbps
DQS_IN_ODTOFF_4266   with no ODT, 3200-4266Mbps
DQS_IN_ODT40_4266   with 40ohm ODT, 3200-4266Mbps
DQS_IN_ODT48_4266   with 48ohm ODT, 3200-4266Mbps
DQS_IN_ODT60_4266   with 60ohm ODT, 3200-4266Mbps
DQS_IN_ODT80_4266   with 80ohm ODT, 3200-4266Mbps
DQS_IN_ODT120_4266   with 120ohm ODT, 3200-4266Mbps
DQS_IN_ODT240_4266   with 240ohm ODT, 3200-4266Mbps
[Model Selector] CA_INPUT
| CA Input models
CA_INPUT_ODTOFF_4266   with no ODT, 3200-4266Mbps
CA_INPUT_ODT40_4266   with 40ohm ODT, 3200-4266Mbps
CA_INPUT_ODT48_4266   with 48ohm ODT, 3200-4266Mbps
CA_INPUT_ODT60_4266   with 60ohm ODT, 3200-4266Mbps
CA_INPUT_ODT80_4266   with 80ohm ODT, 3200-4266Mbps
CA_INPUT_ODT120_4266   with 120ohm ODT, 3200-4266Mbps
CA_INPUT_ODT240_4266   with 240ohm ODT, 3200-4266Mbps
[Model Selector] CS_INPUT
| CS Input models
CS_INPUT_ODTOFF_4266   with no ODT, 3200-4266Mbps
CS_INPUT_ODT40_4266   with 40ohm ODT, 3200-4266Mbps
CS_INPUT_ODT48_4266   with 48ohm ODT, 3200-4266Mbps
CS_INPUT_ODT60_4266   with 60ohm ODT, 3200-4266Mbps
CS_INPUT_ODT80_4266   with 80ohm ODT, 3200-4266Mbps
CS_INPUT_ODT120_4266   with 120ohm ODT, 3200-4266Mbps
CS_INPUT_ODT240_4266   with 240ohm ODT, 3200-4266Mbps
[Model Selector] CLK_INPUT
| Clock Input models
CLK_INPUT_ODTOFF_4266   with no ODT, 3200-4266Mbps
CLK_INPUT_ODT40_4266   with 40ohm ODT, 3200-4266Mbps
CLK_INPUT_ODT48_4266   with 48ohm ODT, 3200-4266Mbps
CLK_INPUT_ODT60_4266   with 60ohm ODT, 3200-4266Mbps
CLK_INPUT_ODT80_4266   with 80ohm ODT, 3200-4266Mbps
CLK_INPUT_ODT120_4266   with 120ohm ODT, 3200-4266Mbps
CLK_INPUT_ODT240_4266   with 240ohm ODT, 3200-4266Mbps
| Models and submodels in the file (175): DQ_PD40_SOC-ODT40_VOH30_4266 (I/O), DQ_PD40_SOC-ODT48_VOH30_4266 (I/O), DQ_PD40_SOC-ODT60_VOH30_4266 (I/O), DQ_PD40_SOC-ODT80_VOH30_4266 (I/O), DQ_PD40_SOC-ODT120_VOH30_4266 (I/O), DQ_PD40_SOC-ODT240_VOH30_4266 (I/O), DQ_PD40_SOC-ODTDIS_VOH30_4266 (I/O), DQ_PD40_SOC-ODT80_VOH25_4266 (I/O), DQ_PD40_SOC-ODT120_VOH25_4266 (I/O), DQ_PD40_SOC-ODT240_VOH25_4266 (I/O), DQ_PD40_SOC-ODTDIS_VOH25_4266 (I/O), DQ_PD48_SOC-ODT40_VOH30_4266 (I/O), DQ_PD48_SOC-ODT48_VOH30_4266 (I/O), DQ_PD48_SOC-ODT60_VOH30_4266 (I/O), DQ_PD48_SOC-ODT80_VOH30_4266 (I/O), DQ_PD48_SOC-ODT120_VOH30_4266 (I/O), DQ_PD48_SOC-ODT240_VOH30_4266 (I/O), DQ_PD48_SOC-ODTDIS_VOH30_4266 (I/O), DQ_PD48_SOC-ODT80_VOH25_4266 (I/O), DQ_PD48_SOC-ODT120_VOH25_4266 (I/O), DQ_PD48_SOC-ODT240_VOH25_4266 (I/O), DQ_PD48_SOC-ODTDIS_VOH25_4266 (I/O), DQ_PD60_SOC-ODT40_VOH30_4266 (I/O), DQ_PD60_SOC-ODT48_VOH30_4266 (I/O), DQ_PD60_SOC-ODT60_VOH30_4266 (I/O), DQ_PD60_SOC-ODT80_VOH30_4266 (I/O), DQ_PD60_SOC-ODT120_VOH30_4266 (I/O), DQ_PD60_SOC-ODT240_VOH30_4266 (I/O), DQ_PD60_SOC-ODTDIS_VOH30_4266 (I/O), DQ_PD60_SOC-ODT80_VOH25_4266 (I/O), DQ_PD60_SOC-ODT120_VOH25_4266 (I/O), DQ_PD60_SOC-ODT240_VOH25_4266 (I/O), DQ_PD60_SOC-ODTDIS_VOH25_4266 (I/O), DQ_PD80_SOC-ODT40_VOH30_4266 (I/O), DQ_PD80_SOC-ODT48_VOH30_4266 (I/O), DQ_PD80_SOC-ODT60_VOH30_4266 (I/O), DQ_PD80_SOC-ODT80_VOH30_4266 (I/O), DQ_PD80_SOC-ODT120_VOH30_4266 (I/O), DQ_PD80_SOC-ODT240_VOH30_4266 (I/O), DQ_PD80_SOC-ODTDIS_VOH30_4266 (I/O), DQ_PD80_SOC-ODT80_VOH25_4266 (I/O), DQ_PD80_SOC-ODT120_VOH25_4266 (I/O), DQ_PD80_SOC-ODT240_VOH25_4266 (I/O), DQ_PD80_SOC-ODTDIS_VOH25_4266 (I/O), DQ_PD120_SOC-ODT40_VOH30_4266 (I/O), DQ_PD120_SOC-ODT48_VOH30_4266 (I/O), DQ_PD120_SOC-ODT60_VOH30_4266 (I/O), DQ_PD120_SOC-ODT80_VOH30_4266 (I/O), DQ_PD120_SOC-ODT120_VOH30_4266 (I/O), DQ_PD120_SOC-ODT240_VOH30_4266 (I/O), DQ_PD120_SOC-ODTDIS_VOH30_4266 (I/O), DQ_PD120_SOC-ODT80_VOH25_4266 (I/O), DQ_PD120_SOC-ODT120_VOH25_4266 (I/O), DQ_PD120_SOC-ODT240_VOH25_4266 (I/O), DQ_PD120_SOC-ODTDIS_VOH25_4266 (I/O), DQ_PD240_SOC-ODT40_VOH30_4266 (I/O), DQ_PD240_SOC-ODT48_VOH30_4266 (I/O), DQ_PD240_SOC-ODT60_VOH30_4266 (I/O), DQ_PD240_SOC-ODT80_VOH30_4266 (I/O), DQ_PD240_SOC-ODT120_VOH30_4266 (I/O), DQ_PD240_SOC-ODT240_VOH30_4266 (I/O), DQ_PD240_SOC-ODTDIS_VOH30_4266 (I/O), DQ_PD240_SOC-ODT80_VOH25_4266 (I/O), DQ_PD240_SOC-ODT120_VOH25_4266 (I/O), DQ_PD240_SOC-ODT240_VOH25_4266 (I/O), DQ_PD240_SOC-ODTDIS_VOH25_4266 (I/O), DQ_IN_ODTOFF_4266 (Input), DQ_IN_ODT40_4266 (Input), DQ_IN_ODT48_4266 (Input), DQ_IN_ODT60_4266 (Input), DQ_IN_ODT80_4266 (Input), DQ_IN_ODT120_4266 (Input), DQ_IN_ODT240_4266 (Input), DQS_PD40_SOC-ODT40_VOH30_4266 (I/O), DQS_PD40_SOC-ODT48_VOH30_4266 (I/O), DQS_PD40_SOC-ODT60_VOH30_4266 (I/O), DQS_PD40_SOC-ODT80_VOH30_4266 (I/O), DQS_PD40_SOC-ODT120_VOH30_4266 (I/O), DQS_PD40_SOC-ODT240_VOH30_4266 (I/O), DQS_PD40_SOC-ODTDIS_VOH30_4266 (I/O)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
